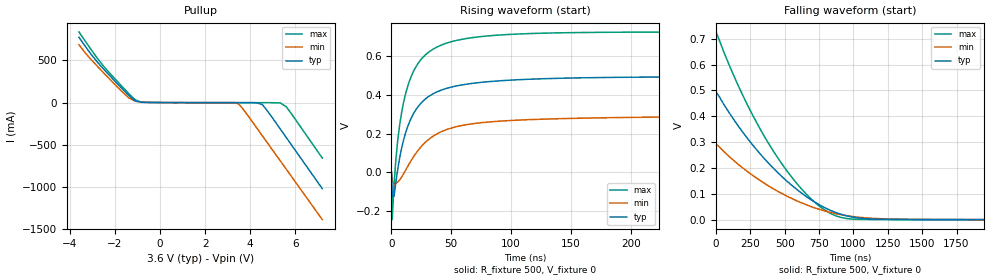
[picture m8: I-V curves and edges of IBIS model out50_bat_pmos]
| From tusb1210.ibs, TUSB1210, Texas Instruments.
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|   Model: out50_bat_pmos
|   Description:  Output buffer under VBAT PMOS enabled
[Model]   out50_bat_pmos
Model_type   Open_source
Polarity   Non-Inverting
Vmeas =   0.500
Vref =   0
Cref =   5e-12
Rref =   2.7e3
|variable   typ   min   max
C_comp   0.087p   0.067p   0.184p
[Temperature Range]   27   125   -40
[Voltage Range]   3.6   2.7   4.5
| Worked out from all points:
|   slope of the pullup table from 0 to 0.54 V, typ, clamps not added: 570 ohm
|   rising waveform, R_fixture 500, V_fixture 0: 20-80 % time 24.2ns typ, 35.4ns min, 19.4ns max; typ from 0 V to 0.494 V
|   falling waveform, R_fixture 500, V_fixture 0: 20-80 % time 514ns typ, 536ns min, 470ns max; typ from 0.495 V to 0 V
[Pullup]
| out50_bat_pmos
|Voltage   I(typ)   I(min)   I(max)
-3.6V     774mA      686mA      837.8mA
-3.045V   567.2mA    505.7mA    622.9mA
-2.49V    393.2mA    348.2mA    425.5mA
-1.38V    82.25mA    54.58mA    104mA
-1.103V   19.41mA    16.33mA    31.43mA
-825mV    2.848mA    5.981mA    3.142mA
3.45V     -989.9uA   -12.69mA   -1.452mA
4.275V    -2.542mA   -296mA     -1.453mA
4.541V    -25.44mA   -395.6mA   -1.454mA
5.339V    -315.9mA   -694.1mA   -4.336mA
5.604V    -417.2mA   -793.6mA   -51.5mA
7.2V      -1.024A    -1.391A    -659.4mA
[Ramp]
| out50_bat_pmos
|variable   typ   min   max
dV/dt_r   0.495/2.724e-08   0.292/3.991e-08   0.726/2.128e-08
dV/dt_f   1.355/7.311e-07   1.082/7.070e-07   1.662/6.895e-07
R_load =   50
[Rising Waveform]
| out50_bat_pmos
R_fixture =   500
V_fixture =   0
V_fixture_min =   0
V_fixture_max =   0
|Time   V(typ)   V(min)   V(max)
0s        755.8nV    12.75uV    673.3nV
644.8ps   -121.9mV   -35.89mV   -245.5mV
2.211ns   -123.8mV   -68.85mV   -65.49mV
5.342ns   17.84mV    -50.02mV   168.4mV
8.474ns   122.6mV    -25.47mV   306.7mV
13.17ns   228.6mV    24.97mV    435.5mV
24.13ns   353.4mV    127.3mV    578.7mV
42.92ns   427.8mV    213.1mV    660.9mV
113.7ns   480.8mV    271.7mV    717.1mV
310.9ns   494.1mV    288.9mV    725.7mV
[Falling Waveform]
| out50_bat_pmos
R_fixture =   500
V_fixture =   0
V_fixture_min =   0
V_fixture_max =   0
|Time   V(typ)   V(min)   V(max)
0s        494.6mV    292.3mV    726.2mV
103.6ns   407.2mV    240.5mV    588.5mV
207.2ns   329.5mV    194.9mV    467.3mV
435.1ns   189.4mV    114mV      250.7mV
663.1ns   87.02mV    56.54mV    95.41mV
787.4ns   47.56mV    34.25mV    38.71mV
870.3ns   27.93mV    23.45mV    15.13mV
1.036us   6.586mV    9.689mV    1.367mV
1.243us   1.119mV    3.07mV     466uV
4.105us   1.08uV     13.18uV    1.013uV
